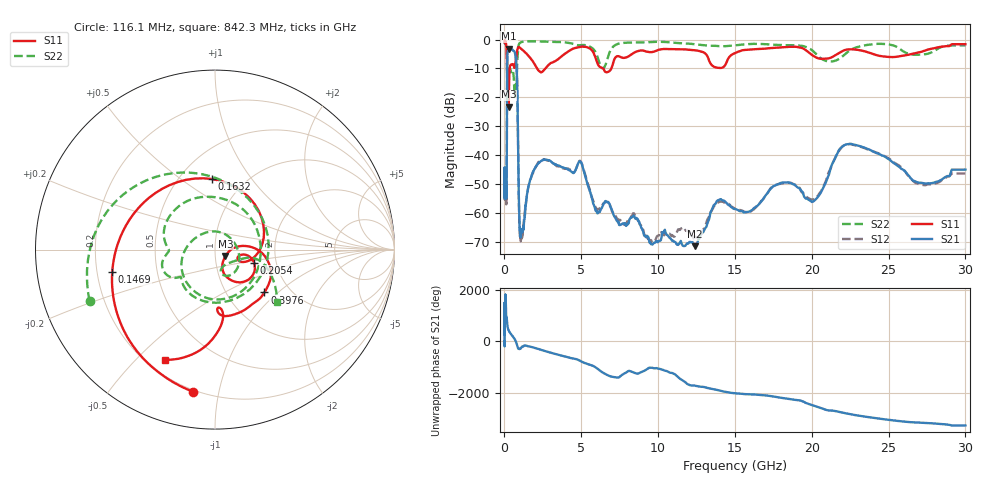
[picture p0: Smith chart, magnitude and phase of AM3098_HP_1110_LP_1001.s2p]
! Date/Time: Thu, Feb 28, 2019 8:46 AM
! Network Analyzer: Agilent Technologies E8364B Rev: A.07.50.67
! Sweep from 0.010 to 30.000 GHz, 1601 Points, Sweep Type: LOG
! Power Supply: 5.022 V, 0.002 A
# Hz S DB R 50
!freq MagS11 AngS11 MagS21 AngS21 MagS12 AngS12 MagS22 AngS22
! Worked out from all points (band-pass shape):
!   1601 points, 10 MHz to 30 GHz, reference 50 ohm
!   highest |S21| = -3.07 dB at 297.5 MHz (marker M1); lowest = -71.6 dB at 12.37 GHz (marker M2)
!   |S21| within 3 dB of the highest: 183.7 MHz to 737 MHz (553.3 MHz wide, 120 % of centre)
!   lowest |S11| = -23.3 dB at 265.1 MHz (marker M3), VSWR 1.15, Z = 56.1 - j4.03 ohm
!   |S11| at or under -10 dB: 169.6 MHz to 340.1 MHz (170.4 MHz wide, 66.9 % of centre); 2.12 GHz to 2.664 GHz (544.2 MHz wide, 22.8 % of centre); 6.414 GHz to 6.957 GHz (543.3 MHz wide, 8.13 % of centre)
!   |S22| runs from -19.9 to -0.5 dB; largest |S21 - S12| = 0.011
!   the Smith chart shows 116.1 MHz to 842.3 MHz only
!   S11 on the Smith chart (normalised r, x): 116.1 MHz: 0.19, -0.84; 146.9 MHz: 0.26, -0.10; 163.2 MHz: 0.71, +0.66; 205.4 MHz: 1.53, -0.24; 397.6 MHz: 1.49, -0.82; 842.3 MHz: 0.27, -0.61
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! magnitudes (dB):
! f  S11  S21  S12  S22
! 10 MHz  -0.4  -45.9  -44.6  -0.6
! 38.04 MHz  -0.3  -50.2  -50.4  -0.8
! 116.1 MHz  -1.9  -53.1  -54.4  -2.4
! 144.7 MHz  -4.3  -50.4  -51.6  -5.5
! 146.9 MHz  -4.6  -48.0  -49.0  -6.0
! 163.2 MHz  -8.1  -21.0  -20.9  -10.6
! 205.4 MHz  -12.8  -4.2  -4.2  -10.7
! 265.1 MHz  -23.3  -3.1  -3.1  -11.8
! 297.5 MHz  -14.9  -3.1  -3.0  -11.3
! 397.6 MHz  -8.8  -3.2  -3.2  -10.5
! 550.5 MHz  -8.5  -3.7  -3.7  -11.1
! 765.9 MHz  -6.0  -7.6  -7.6  -19.7
! 842.3 MHz  -3.4  -18.7  -18.7  -6.9
! 949.8 MHz  -2.6  -57.9  -59.5  -1.5
! 1.029 GHz  -2.9  -67.7  -69.0  -1.0
! 2.084 GHz  -9.6  -43.7  -43.8  -0.6
! 4.927 GHz  -2.5  -42.3  -42.0  -1.9
! 7.926 GHz  -6.2  -64.6  -63.7  -1.1
! 12.37 GHz  -3.7  -71.6  -68.4  -1.6
! 20.2 GHz  -6.0  -55.6  -55.3  -4.5
! 22.56 GHz  -3.3  -36.1  -36.3  -3.5
! 30 GHz  -1.6  -45.1  -46.4  -2.0
